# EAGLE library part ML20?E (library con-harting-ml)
HARTING
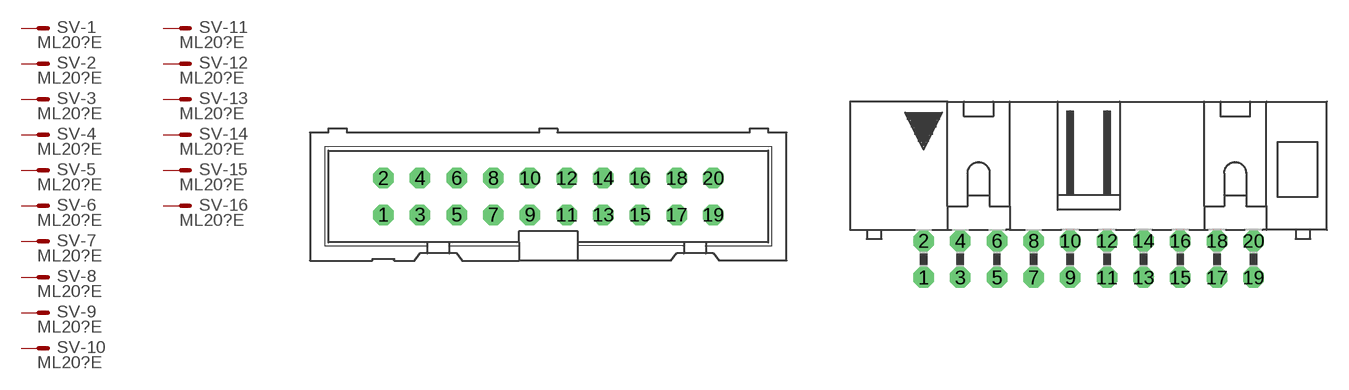
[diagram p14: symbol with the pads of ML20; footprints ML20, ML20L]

Designator prefix SV; gates -1=M -2=M -3=M -4=M -5=M -6=M -7=M -8=M -9=M -10=M -11=M -12=M -13=M -14=M -15=M -16=M -17=M -18=M -19=M -20=M

## ML20E (OC_FARNELL: unknown; OC_NEWARK: unknown)  [ML20]
1  -1:S  pas
2  -2:S  pas
3  -3:S  pas
4  -4:S  pas
5  -5:S  pas
6  -6:S  pas
7  -7:S  pas
8  -8:S  pas
9  -9:S  pas
10  -10:S  pas
11  -11:S  pas
12  -12:S  pas
13  -13:S  pas
14  -14:S  pas
15  -15:S  pas
16  -16:S  pas
17  -17:S  pas
18  -18:S  pas
19  -19:S  pas
20  -20:S  pas

## ML20LE (OC_FARNELL: unknown; OC_NEWARK: unknown)  [ML20L]
Pads as for ML20

## ML203ME (OC_FARNELL: unknown; OC_NEWARK: unknown)  [3M_20]
Pads as for ML20

## ML203M20LE (OC_FARNELL: unknown; OC_NEWARK: unknown)  [3M_20L]
Pads as for ML20

## Footprint ML20 (pad centres in mm)
HARTING
drill 0.914 octagon: 1 -11.43,-1.27; 2 -11.43,1.27; 3 -8.89,-1.27; 4 -8.89,1.27; 5 -6.35,-1.27; 6 -6.35,1.27; 7 -3.81,-1.27; 8 -3.81,1.27; 9 -1.27,-1.27; 10 -1.27,1.27; 11 1.27,-1.27; 12 1.27,1.27; 13 3.81,-1.27; 14 3.81,1.27; 15 6.35,-1.27; 16 6.35,1.27; 17 8.89,-1.27; 18 8.89,1.27; 19 11.43,-1.27; 20 11.43,1.27

## Footprint ML20L (pad centres in mm)
HARTING
drill 0.914 octagon: 1 -11.43,-1.27; 2 -11.43,1.27; 3 -8.89,-1.27; 4 -8.89,1.27; 5 -6.35,-1.27; 6 -6.35,1.27; 7 -3.81,-1.27; 8 -3.81,1.27; 9 -1.27,-1.27; 10 -1.27,1.27; 11 1.27,-1.27; 12 1.27,1.27; 13 3.81,-1.27; 14 3.81,1.27; 15 6.35,-1.27; 16 6.35,1.27; 17 8.89,-1.27; 18 8.89,1.27; 19 11.43,-1.27; 20 11.43,1.27

## Footprint 3M_20 (pad centres in mm)
3M
drill 0.813 square: 1 -11.43,-1.27; 2 -11.43,1.27; 3 -8.89,-1.27; 4 -8.89,1.27; 5 -6.35,-1.27; 6 -6.35,1.27; 7 -3.81,-1.27; 8 -3.81,1.27; 9 -1.27,-1.27; 10 -1.27,1.27; 11 1.27,-1.27; 12 1.27,1.27; 13 3.81,-1.27; 14 3.81,1.27; 15 6.35,-1.27; 16 6.35,1.27; 17 8.89,-1.27; 18 8.89,1.27; 19 11.43,-1.27; 20 11.43,1.27

## Footprint 3M_20L (pad centres in mm)
3M
drill 0.813 square: 1 -11.43,-5.08; 2 -11.43,-2.54; 3 -8.89,-5.08; 4 -8.89,-2.54; 5 -6.35,-5.08; 6 -6.35,-2.54; 7 -3.81,-5.08; 8 -3.81,-2.54; 9 -1.27,-5.08; 10 -1.27,-2.54; 11 1.27,-5.08; 12 1.27,-2.54; 13 3.81,-5.08; 14 3.81,-2.54; 15 6.35,-5.08; 16 6.35,-2.54; 17 8.89,-5.08; 18 8.89,-2.54; 19 11.43,-5.08; 20 11.43,-2.54
hole 2.54 at -17.348,-3.277
hole 2.54 at 17.348,-3.277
